{attribute 'qualified_only'}
VAR_GLOBAL PERSISTENT
	// Persistant calculated damage of former runs read from file.
	fDamage_RFC		: LREAL;		// Persistant damage
	fDamage_MSC		: LREAL;		// Persistant damage
	nCycles_RFC		: ULINT;		// Persistant number of cycles counted
	nCycles_MSC		: ULINT;		// Persistant number of cycles counted
END_VAR
